FUNCTION_BLOCK CheckXbotState	//Rising edge triggered wrapper of the ReadXbotState command
VAR_INPUT
	Execute : BOOL;	// Execution of the function block begins on a rising edge of this input.
	XbotID : USINT;	// xbot ID# (1-78)
END_VAR
VAR_OUTPUT
	Done : BOOL;	// Execution successful. Function block is finished
	Valid : BOOL;	// successfully read xbot state
	State : USINT;   // 0 = undetected, 1 = discovering, 2 = landed, 3 = idle, 4 = disabled, 5 = in motion, 6 = waiting, 7 = stopping, 8 = obstacle, 9 = hold, 10 = stopped, 14 = error
END_VAR
VAR_IN_OUT
	PM_Controller : PMControllerType;	// the planar motor controller to use
END_VAR
VAR
	ReadXbotState : PMC_ReadXbotState;
END_VAR

IF(Execute = FALSE)THEN
	Done := FALSE;
	ReadXbotState(Enable := FALSE,PM_Controller := PM_Controller);
END_IF;

IF(Execute = TRUE AND Done = FALSE)THEN
	Done := TRUE;
	ReadXbotState(Enable := TRUE,XbotID := XbotID,Valid => Valid,State => State,PM_Controller := PM_Controller);
END_IF;

END_FUNCTION_BLOCK
